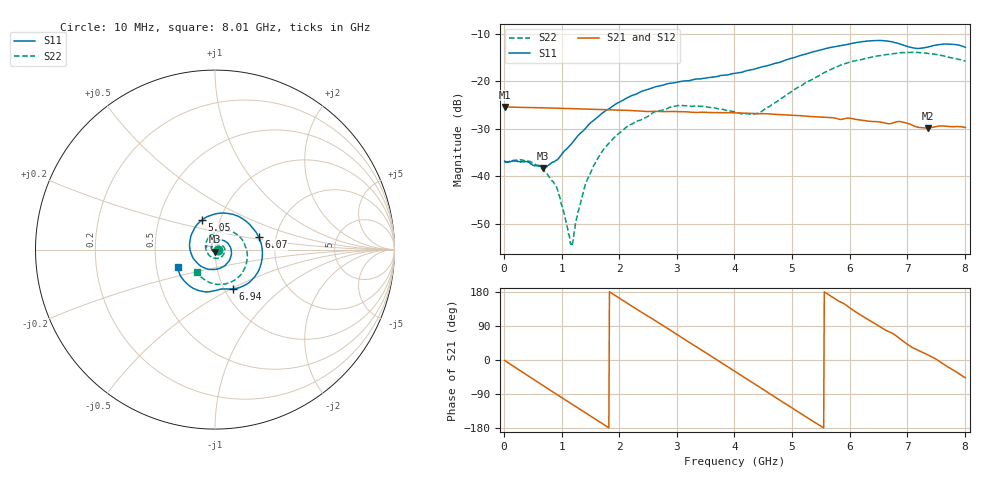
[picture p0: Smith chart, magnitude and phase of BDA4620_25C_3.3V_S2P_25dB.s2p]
!Agilent Technologies,E5071B,MY42404982,A.09.10
!Date: Wed May 06 08:54:15 2026
!Data & Calibration Information:
!Freq	S11:SOLT2(ON)	S21:SOLT2(ON)	S12:SOLT2(ON)	S22:SOLT2(ON)
# Hz S RI R 50
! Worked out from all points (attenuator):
!   801 points, 10 MHz to 8.01 GHz, reference 50 ohm
!   highest |S21| = -25.39 dB at 10 MHz (marker M1); lowest = -29.8 dB at 7.36 GHz (marker M2)
!   lowest |S11| = -38.3 dB at 680 MHz (marker M3), VSWR 1.02, Z = 49.8 - j1.19 ohm
!   |S11| at or under -10 dB: start of sweep to end of sweep
!   |S22| runs from -54.7 to -13.9 dB; largest |S21 - S12| = 0.00027
!   S11 on the Smith chart (normalised r, x): 10 MHz: 1.03, -0.00; 5.05 GHz: 0.82, +0.28; 6.07 GHz: 1.62, +0.25; 6.94 GHz: 1.09, -0.51; 8.01 GHz: 0.65, -0.13
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1e7  0.0144 -0.00095  0.0538 -0.00113  0.0539 -0.00113  0.0141 -0.000461
4.2e8  0.00853 -0.0112  0.0394 -0.0354  0.0395 -0.0355  0.0136 -0.00493
6.8e8  -0.002 -0.012  0.02 -0.0486  0.02 -0.0488  0.00935 -0.00695
9.3e8  -0.0138 -0.00585  -0.00203 -0.0521  -0.00209 -0.0522  0.00352 -0.00625
1.16e9  -0.0203 0.00715  -0.0217 -0.0468  -0.0217 -0.0469  -0.00153 -0.00117
1.2e9  -0.0209 0.00993  -0.0248 -0.0452  -0.0248 -0.0452  -0.00212 5.26e-06
1.35e9  -0.0207 0.0208  -0.0352 -0.0372  -0.0352 -0.0372  -0.00365 0.0046
1.53e9  -0.015 0.0347  -0.0444 -0.0247  -0.0444 -0.0247  -0.00347 0.0113
1.77e9  0.00157 0.0493  -0.05 -0.00506  -0.0501 -0.00505  0.000648 0.0206
2.15e9  0.0422 0.0529  -0.0423 0.0256  -0.0423 0.0256  0.017 0.0294
2.68e9  0.0891 0.00459  -0.00704 0.0477  -0.00699 0.0477  0.0444 0.0195
3.08e9  0.0813 -0.0584  0.0241 0.0414  0.0243 0.0414  0.0553 -0.00735
4.01e9  -0.0832 -0.0888  0.0403 -0.0233  0.0404 -0.0234  -0.0104 -0.0467
4.42e9  -0.1388 -0.00163  0.0158 -0.0429  0.0158 -0.0429  -0.0445 -0.0128
5.05e9  -0.073 0.1636  -0.0289 -0.0329  -0.029 -0.033  -0.0253 0.0784
5.35e9  0.0209 0.2024  -0.0401 -0.0144  -0.0401 -0.0144  0.0228 0.1021
6.07e9  0.2429 0.0717  -0.026 0.0307  -0.0261 0.0307  0.1562 0.0484
6.68e9  0.1932 -0.1807  0.00945 0.0345  0.00948 0.0346  0.1705 -0.0903
6.94e9  0.0979 -0.2193  0.0247 0.0276  0.0248 0.0276  0.1371 -0.1474
7.36e9  -0.00687 -0.2297  0.0313 0.00757  0.0315 0.00758  0.0376 -0.1934
7.66e9  -0.1192 -0.2169  0.0327 -0.00802  0.0328 -0.00808  -0.0357 -0.1803
8.01e9  -0.2077 -0.0952  0.0222 -0.0239  0.0222 -0.0239  -0.1021 -0.1275
